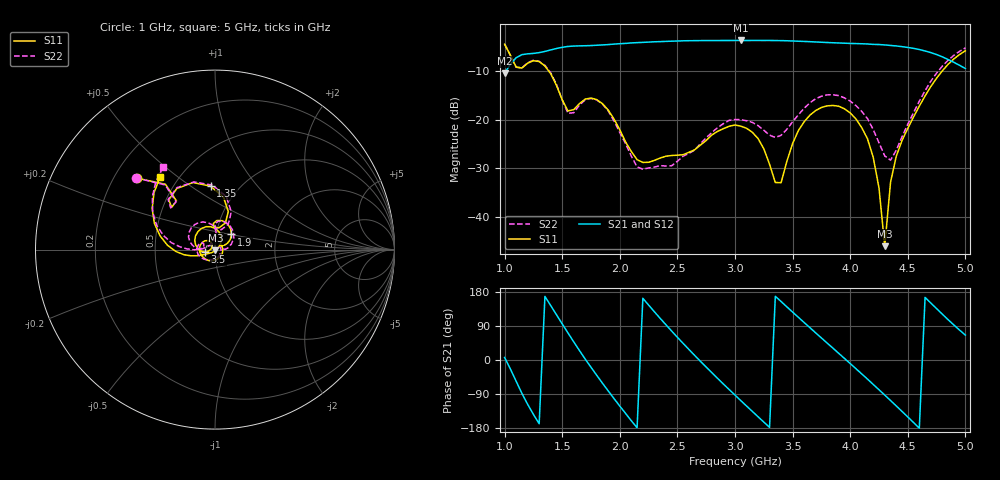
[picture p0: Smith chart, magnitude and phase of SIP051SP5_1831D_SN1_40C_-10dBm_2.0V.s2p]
# GHz  S  dB  R  50
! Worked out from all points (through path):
!   81 points, 1 GHz to 5 GHz, reference 50 ohm
!   highest |S21| = -3.79 dB at 3.05 GHz (marker M1); lowest = -10.5 dB at 1 GHz (marker M2)
!   lowest |S11| = -45.9 dB at 4.3 GHz (marker M3), VSWR 1.01, Z = 50.2 - j0.474 ohm
!   |S11| at or under -10 dB: 1.381 GHz to 4.8 GHz (3.419 GHz wide, 111 % of centre)
!   |S22| runs from -30.2 to -4.5 dB; largest |S21 - S12| = 0.0031
!   S11 on the Smith chart (normalised r, x): 1 GHz: 0.29, +0.36; 1.35 GHz: 0.74, +0.60; 1.9 GHz: 1.18, +0.20; 3.5 GHz: 0.89, -0.02; 5 GHz: 0.40, +0.43
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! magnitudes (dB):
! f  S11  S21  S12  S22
! 1 GHz  -4.6  -10.5  -10.5  -4.5
! 1.1 GHz  -9.2  -7.3  -7.3  -9.3
! 1.35 GHz  -9.0  -6.0  -6.0  -8.9
! 1.55 GHz  -18.2  -5.0  -5.0  -18.7
! 1.7 GHz  -15.8  -4.9  -4.9  -15.9
! 1.9 GHz  -18.1  -4.6  -4.6  -18.2
! 2.15 GHz  -28.2  -4.2  -4.2  -29.7
! 2.35 GHz  -27.9  -4.0  -4.0  -29.4
! 3 GHz  -21.1  -3.8  -3.8  -20.0
! 3.05 GHz  -21.3  -3.8  -3.8  -20.0
! 3.2 GHz  -23.9  -3.8  -3.8  -21.2
! 3.35 GHz  -32.9  -3.8  -3.8  -23.7
! 3.4 GHz  -32.9  -3.8  -3.8  -23.2
! 3.5 GHz  -24.9  -3.9  -3.9  -20.4
! 3.7 GHz  -18.2  -4.1  -4.1  -15.7
! 3.95 GHz  -17.8  -4.3  -4.4  -15.5
! 4.15 GHz  -23.9  -4.5  -4.5  -19.8
! 4.25 GHz  -34.0  -4.6  -4.6  -24.8
! 4.3 GHz  -45.9  -4.7  -4.7  -27.5
! 4.35 GHz  -32.9  -4.8  -4.8  -28.3
! 4.65 GHz  -15.1  -5.9  -5.9  -14.1
! 5 GHz  -5.9  -9.5  -9.5  -5.3
